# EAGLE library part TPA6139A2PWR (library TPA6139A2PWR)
DirectPath 25mW Headphone Amplifier Source: Datasheet
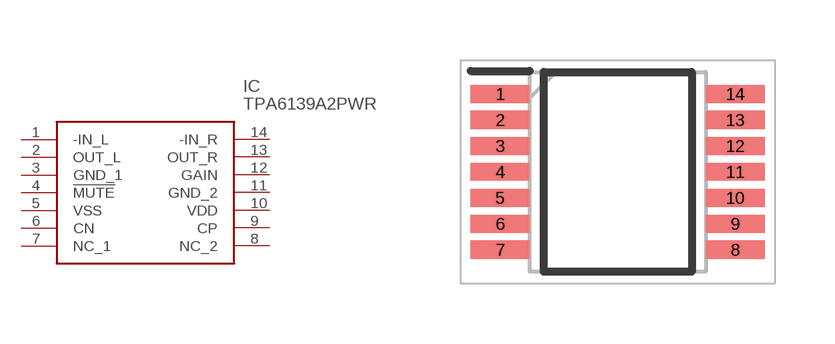
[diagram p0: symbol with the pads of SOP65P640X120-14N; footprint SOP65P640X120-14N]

Designator prefix IC

## TPA6139A2PWR (Arrow_Part_Number: TPA6139A2PWR; Arrow_Price-Stock: https://www.arrow.com/en/products/tpa6139a2pwr/texas-instruments?region=nac; Description: DirectPath 25mW Headphone Amplifier; Height: 1.2mm; Manufacturer_Name: Texas Instruments; Manufacturer_Part_Number: TPA6139A2PWR; Mouser_Part_Number: 595-TPA6139A2PWR; Mouser_Price-Stock: https://www.mouser.co.uk/ProductDetail/Texas-Instruments/TPA6139A2PWR?qs=TeC8nwD7mVr7iydXyN4ieA%3D%3D)  [SOP65P640X120-14N]
1  -IN_L
2  OUT_L
3  GND_1
4  !MUTE
5  VSS
6  CN
7  NC_1
8  NC_2
9  CP
10  VDD
11  GND_2
12  GAIN
13  OUT_R
14  -IN_R

## Footprint SOP65P640X120-14N (pad centres in mm)
PW
smd 1.475 x 0.45: 1 -2.938,1.95; 2 -2.938,1.3; 3 -2.938,0.65; 4 -2.938,0; 5 -2.938,-0.65; 6 -2.938,-1.3; 7 -2.938,-1.95; 8 2.938,-1.95; 9 2.938,-1.3; 10 2.938,-0.65; 11 2.938,0; 12 2.938,0.65; 13 2.938,1.3; 14 2.938,1.95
